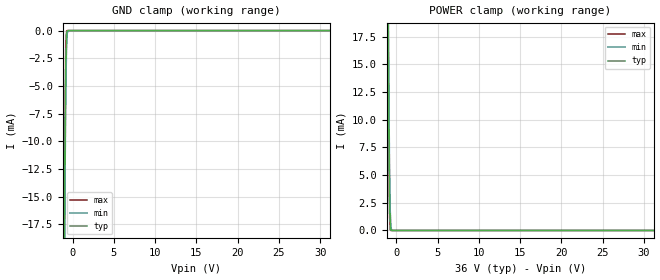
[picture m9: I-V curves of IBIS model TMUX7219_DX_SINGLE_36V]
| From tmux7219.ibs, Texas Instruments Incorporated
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[Model]   TMUX7219_DX_SINGLE_36V
Model_type   Terminator
|   typ   min   max
C_comp   47pF   47pF   47pF
[Voltage Range]   30   27   33
[Temperature Range]   27   130   -40
[Power Clamp Reference]   36   32.4   39.6
[GND Clamp Reference]   0   0   0
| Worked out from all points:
|   GND clamp passes 1 mA (typ) near -0.77 V on its own axis
|   POWER clamp passes 1 mA (typ) near -0.77 V on its own axis
[GND Clamp]
|   Voltage   I(typ)   I(min)   I(max)
-30V      -4.646A    -4.808A    -4.649A
-1.02V    -22.01mA   -24.41mA   -19.81mA
-930mV    -11.04mA   -13.89mA   -8.565mA
-840mV    -3.269mA   -5.934mA   -1.414mA
-750mV    -384.6uA   -1.761mA   -36.1uA
-660mV    -13.98uA   -270.8uA   -471.5nA
-570mV    -402.9nA   -19.98uA   -235.8nA
-210mV    0A         0A         0A
60V       0A         0A         0A
[POWER Clamp]
|   Voltage   I(typ)   I(min)   I(max)
-30V      4.646A     4.808A     4.649A
-1.02V    22.01mA    24.41mA    19.81mA
-930mV    11.04mA    13.89mA    8.565mA
-840mV    3.269mA    5.934mA    1.414mA
-750mV    384.6uA    1.761mA    36.1uA
-660mV    13.98uA    270.8uA    471.5nA
-570mV    402.9nA    19.98uA    235.8nA
-210mV    0A         0A         0A
60V       0A         0A         0A
